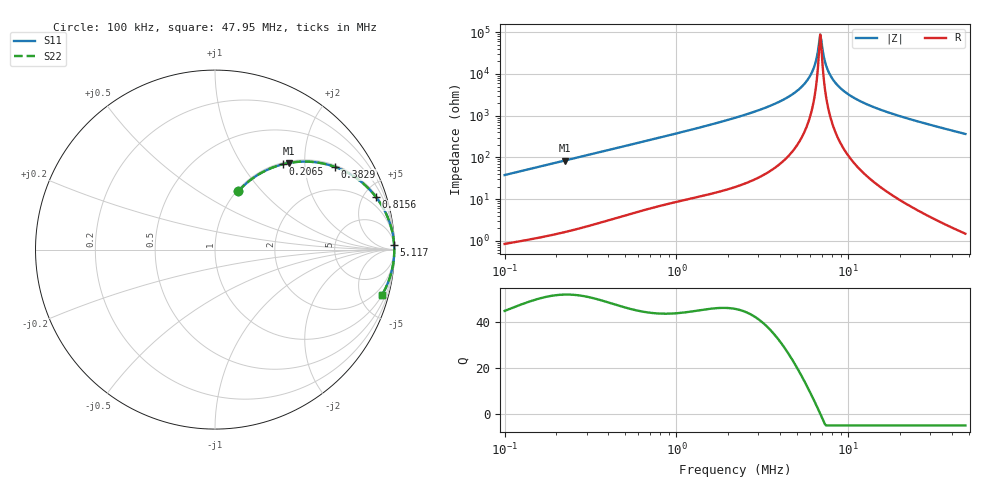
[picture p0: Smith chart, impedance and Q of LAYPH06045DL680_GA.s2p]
! LAYPH06045DL680_GA  S-PARAMETER MODEL  ( General Type )
! Model Generated by TAIYO YUDEN Corporation (http://www.ty-top.com)
! Version 2.0
! TAIYO YUDEN Control No. 180914NI43SB-FBB
! Copyright(c) 2018 TAIYO YUDEN CO.,LTD. All Rights Reserved.
! Product Description (link to TY-COMPAS)
! https://ds.yuden.co.jp/TYCOMPAS/or/detail?pn=LAYPH06045DL680MGA&u=M
! Products Name : Inductors
! Characteristics :
!  Inductance : 68 uH , SRF(min) : -Hz , DC Resistance(max) : 0.252 Ohm
!  Rated Current : Saturation :0.8 A , Temp Rise : 0.73 A (25 degC)
!  Case Size : 6.3 x 6.0 / 0.248 x 0.236 [mm/inch] , Thickness : 4.5 / 0.177 [mm/inch]
!  (Conditions: Temperature = 25 degC , DC Bias Current/Voltage = 0A / 0V)
! External Node Assignments :
!  1  o---GGG---o  2
! GND o---------o GND
! Frequency Range : 0.1MHz  -  47.953651MHz  [ 402 STEP ]
# MHz S RI R 50
! Freq[MHz].  S11 Real  S11 Imag  S21 Real  S21 Imag  S12 Real  S12 Imag  S22 Real  S22 Imag
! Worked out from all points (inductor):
!   401 points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, 100 kHz to 47.95 MHz, reference 50 ohm
!   read as one part in series: L = 60 uH near 103.1 kHz
!   highest Q = 51.8 at 223.1 kHz (marker M1), where L = 59.8 uH
!   self-resonance near 6.861 MHz
!   S11 on the Smith chart (normalised r, x): 100 kHz: 1.02, +0.76; 206.5 kHz: 1.03, +1.55; 382.9 kHz: 1.06, +2.87; 815.6 kHz: 1.14, +6.11; 5.117 MHz: 5, +83; 47.95 MHz: 1.03, -7.30
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0.1  0.1306 0.326  0.8694 -0.326  0.8694 -0.326  0.1306 0.326
0.206536  0.3783 0.4754  0.6217 -0.4754  0.6217 -0.4754  0.3783 0.4754
0.223104  0.4143 0.483  0.5857 -0.483  0.5857 -0.483  0.4143 0.483
0.281214  0.5263 0.4897  0.4737 -0.4897  0.4737 -0.4897  0.5263 0.4897
0.382894  0.6696 0.4602  0.3304 -0.4602  0.3304 -0.4602  0.6696 0.4602
0.790816  0.8921 0.299  0.1079 -0.299  0.1079 -0.299  0.8921 0.299
0.815604  0.8978 0.2917  0.1022 -0.2917  0.1022 -0.2917  0.8978 0.2917
2.223888  0.9856 0.1086  0.0144 -0.1086  0.0144 -0.1086  0.9856 0.1086
3.700673  0.9957 0.0524  0.00428 -0.0524  0.00428 -0.0524  0.9957 0.0524
5.117099  0.9982 0.0239  0.00183 -0.0239  0.00183 -0.0239  0.9982 0.0239
5.700831  0.9986 0.015  0.00142 -0.015  0.00142 -0.015  0.9986 0.015
6.158125  0.9988 0.00877  0.00124 -0.00877  0.00124 -0.00877  0.9988 0.00877
6.449925  0.9988 0.00505  0.00117 -0.00505  0.00117 -0.00505  0.9988 0.00505
6.755551  0.9989 0.00135  0.00113 -0.00135  0.00113 -0.00135  0.9989 0.00135
6.860612  0.9989 0.000115  0.00112 -0.000115  0.00112 -0.000115  0.9989 0.000115
7.07566  0.9989 -0.00235  0.00112 0.00235  0.00112 0.00235  0.9989 -0.00235
7.297449  0.9989 -0.00482  0.00113 0.00482  0.00113 0.00482  0.9989 -0.00482
7.643235  0.9988 -0.00854  0.00116 0.00854  0.00116 0.00854  0.9988 -0.00854
8.782046  0.9985 -0.0198  0.00145 0.0198  0.00145 0.0198  0.9985 -0.0198
11.41644  0.9972 -0.0423  0.00282 0.0423  0.00282 0.0423  0.9972 -0.0423
17.31754  0.9918 -0.0844  0.00817 0.0844  0.00817 0.0844  0.9918 -0.0844
47.95365  0.9292 -0.2544  0.0708 0.2544  0.0708 0.2544  0.9292 -0.2544
